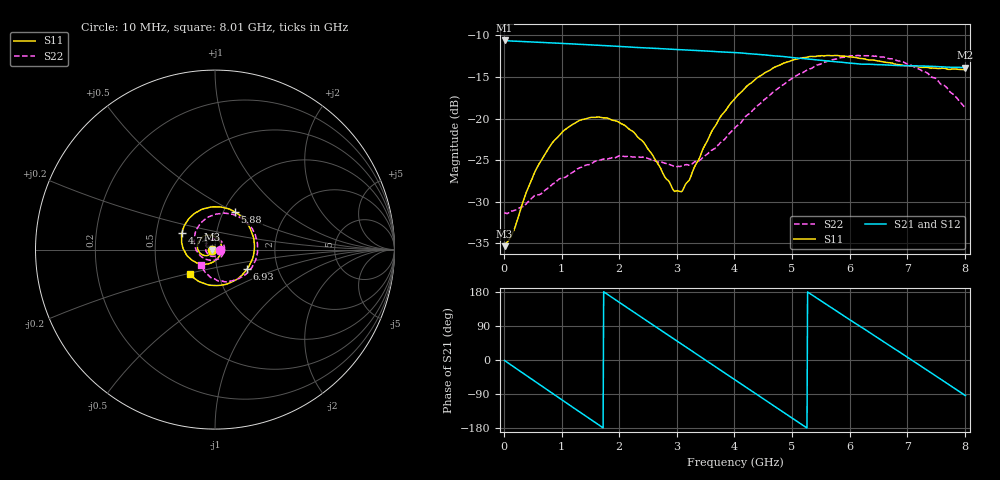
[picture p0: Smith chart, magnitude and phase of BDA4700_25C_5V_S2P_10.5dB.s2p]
!Agilent Technologies,E5071B,MY42404982,A.09.10
!Date: Mon Oct 20 13:31:19 2025
!Data & Calibration Information:
!Freq	S11:SOLT2(ON)	S21:SOLT2(ON)	S12:SOLT2(ON)	S22:SOLT2(ON)
# Hz S RI R 50
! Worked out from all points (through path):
!   801 points, 10 MHz to 8.01 GHz, reference 50 ohm
!   highest |S21| = -10.61 dB at 10 MHz (marker M1); lowest = -13.9 dB at 8.01 GHz (marker M2)
!   group delay of S21, straight-line fit = 282 ps
!   lowest |S11| = -35.3 dB at 10 MHz (marker M3), VSWR 1.03, Z = 48.3 - j0.115 ohm
!   |S11| at or under -10 dB: start of sweep to end of sweep
!   |S22| runs from -31.4 to -12.4 dB; largest |S21 - S12| = 0.0021
!   S11 on the Smith chart (normalised r, x): 10 MHz: 0.97, -0.00; 4.74 GHz: 0.68, +0.13; 5.88 GHz: 1.13, +0.50; 6.93 GHz: 1.39, -0.32; 8.01 GHz: 0.73, -0.21
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1e7  -0.0171 -0.00119  0.2946 -0.00644  0.2945 -0.0067  0.0273 -0.00144
1.6e8  -0.0183 -0.0102  0.2791 -0.0862  0.279 -0.0862  0.0264 -0.00914
3.3e8  -0.0239 -0.0206  0.2377 -0.1665  0.2376 -0.1667  0.0221 -0.0197
7.2e8  -0.0519 -0.0335  0.0708 -0.2771  0.0707 -0.2772  -0.00225 -0.0371
1.02e9  -0.0804 -0.0225  -0.0817 -0.2707  -0.0817 -0.2708  -0.0293 -0.0328
1.35e9  -0.098 0.00982  -0.2165 -0.176  -0.2166 -0.1761  -0.0508 -0.00501
1.93e9  -0.0646 0.0726  -0.2548 0.0956  -0.2547 0.0956  -0.0247 0.0527
2.32e9  -0.0131 0.0763  -0.132 0.2325  -0.132 0.2326  0.0212 0.0548
2.68e9  0.0266 0.0457  0.0323 0.2615  0.0323 0.2615  0.0505 0.0214
2.94e9  0.0363 0.00793  0.1437 0.2175  0.1437 0.217  0.0506 -0.0106
3.09e9  0.0331 -0.0157  0.195 0.1708  0.1942 0.1711  0.0427 -0.0293
3.54e9  -0.018 -0.0725  0.2536 -0.0196  0.2536 -0.0198  -0.0106 -0.0607
4.01e9  -0.1131 -0.0679  0.1524 -0.1971  0.1524 -0.1969  -0.0806 -0.0351
4.37e9  -0.1729 -0.00464  0.00431 -0.2438  0.00412 -0.244  -0.1143 0.0255
4.74e9  -0.1837 0.0941  -0.1425 -0.19  -0.142 -0.1906  -0.1044 0.1075
5.35e9  -0.0617 0.2279  -0.2241 0.0339  -0.2243 0.0333  0.0245 0.1998
5.88e9  0.1119 0.2087  -0.1035 0.1916  -0.1035 0.1912  0.1761 0.1526
6.29e9  0.2013 0.1038  0.0428 0.2076  0.0444 0.2067  0.2359 0.0358
6.68e9  0.2144 -0.0322  0.1617 0.1329  0.1623 0.1327  0.2143 -0.0823
6.93e9  0.1781 -0.1093  0.2009 0.053  0.2012 0.0522  0.1678 -0.1409
7.47e9  0.0213 -0.1999  0.1589 -0.1306  0.1586 -0.1311  0.02 -0.1747
8.01e9  -0.1402 -0.1386  -0.0144 -0.202  -0.0141 -0.2023  -0.0781 -0.0849
